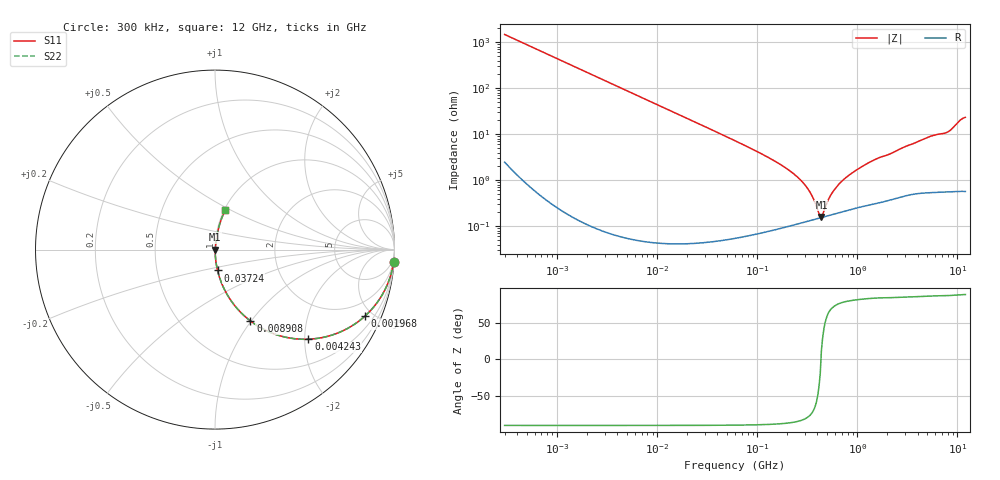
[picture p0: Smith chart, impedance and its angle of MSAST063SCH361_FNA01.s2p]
! MSAST063SCH361_FNA01  S-PARAMETER MODEL  ( General Type )
! Model Generated by TAIYO YUDEN Corporation (http://www.ty-top.com)
! Version 1.0
! TAIYO YUDEN Control No. 160830
! Copyright(c) 2016 TAIYO YUDEN CO.,LTD. All Rights Reserved.
! Product Description (link to TY-COMPAS)
! https://ds.yuden.co.jp/TYCOMPAS/or/detail?pn=MSAST063SCH361JFNA01&u=M
! Products Name : Multilayer Ceramic Capacitors
! Characteristics :
!  Capacitance : 360 pF , Rated Voltage : 25V , TCC : CH / C0H
!  Case Size : 0.6 x 0.3 / 0.024 x 0.012 [mm/inch] , Thickness : 0.3 / 0.012 [mm/inch]
!  (Conditions: Temperature = 25 degC , DC Bias Current/Voltage = 0A / 0V)
! External Node Assignments :
!  1  o---| |---o  2
! GND o---------o GND
! Frequency Range : 0.3MHz  -  12000MHz  [ 401 STEP ]
# MHz S RI R 50
! Freq[MHz].  S11 Real  S11 Imag  S21 Real  S21 Imag  S12 Real  S12 Imag  S22 Real  S22 Imag
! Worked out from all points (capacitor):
!   401 points, 300 kHz to 12 GHz, reference 50 ohm
!   read as one part in series: C = 360 pF near 316.3 kHz
!   lowest |Z| = 158 mohm at 437.6 MHz (marker M1)
!   series resonance near 433.2 MHz, so ESL is about 370 pH
!   S11 on the Smith chart (normalised r, x): 300 kHz: 1, -29; 1.968 MHz: 1.00, -4.49; 4.243 MHz: 1.00, -2.08; 8.908 MHz: 1.00, -0.99; 37.24 MHz: 1.00, -0.24; 12 GHz: 1.01, +0.47
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0.3  0.9953 -0.0675  0.0047 0.0675  0.0047 0.0675  0.9953 -0.0675
0.888858  0.961 -0.1932  0.039 0.1932  0.039 0.1932  0.961 -0.1932
1.769972  0.8617 -0.3449  0.1383 0.3449  0.1383 0.3449  0.8617 -0.3449
1.967827  0.8345 -0.3714  0.1655 0.3714  0.1655 0.3714  0.8345 -0.3714
4.242641  0.5205 -0.4993  0.4795 0.4993  0.4795 0.4993  0.5205 -0.4993
8.908005  0.1977 -0.3978  0.8023 0.3978  0.8023 0.3978  0.1977 -0.3978
10.44266  0.1521 -0.3586  0.8479 0.3586  0.8479 0.3586  0.1521 -0.3586
17.7384  0.0586 -0.2341  0.9414 0.2341  0.9414 0.2341  0.0586 -0.2341
37.24419  0.0141 -0.1161  0.9859 0.1161  0.9859 0.1161  0.0141 -0.1161
60  0.00574 -0.0718  0.9943 0.0718  0.9943 0.0718  0.00574 -0.0718
208.3979  0.00127 -0.0164  0.9987 0.0164  0.9987 0.0164  0.00127 -0.0164
286.3882  0.00128 -0.0088  0.9987 0.0088  0.9987 0.0088  0.00128 -0.0088
353.9943  0.00138 -0.0043  0.9986 0.0043  0.9986 0.0043  0.00138 -0.0043
414.98  0.0015 -0.00107  0.9985 0.00107  0.9985 0.00107  0.0015 -0.00107
437.5599  0.00155 0.000331  0.9985 -0.000331  0.9985 -0.000331  0.00155 0.000331
555.3718  0.00181 0.00484  0.9982 -0.00484  0.9982 -0.00484  0.00181 0.00484
723.8279  0.00218 0.00995  0.9978 -0.00995  0.9978 -0.00995  0.00218 0.00995
1229.528  0.00328 0.0222  0.9967 -0.0222  0.9967 -0.0222  0.00328 0.0222
2088.533  0.00499 0.0364  0.995 -0.0364  0.995 -0.0364  0.00499 0.0364
5140.631  0.0128 0.0857  0.9872 -0.0857  0.9872 -0.0857  0.0128 0.0857
7854.144  0.0172 0.1072  0.9828 -0.1072  0.9828 -0.1072  0.0172 0.1072
12000  0.0563 0.2185  0.9437 -0.2185  0.9437 -0.2185  0.0563 0.2185
